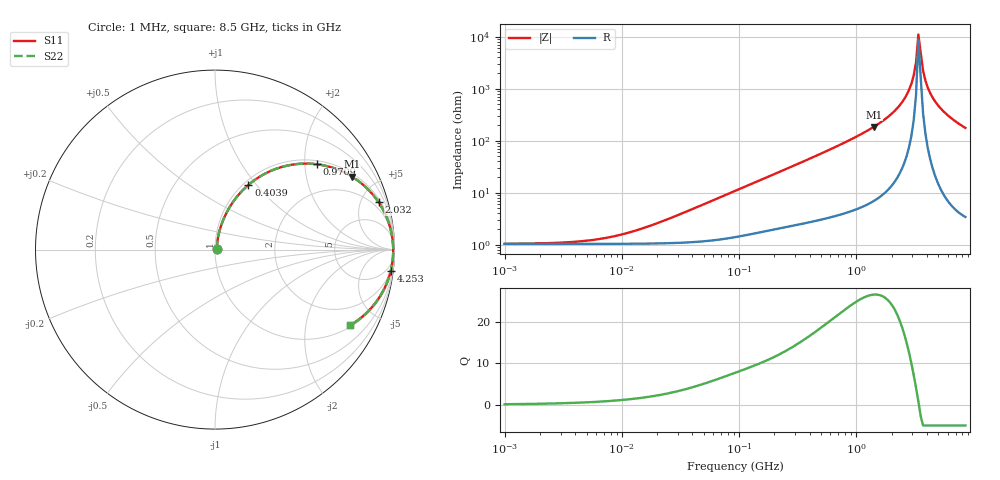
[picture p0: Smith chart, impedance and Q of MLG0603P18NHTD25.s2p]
! S-Parameter Data Generated by TDK Corporation
! Copyright(C) 2025 TDK Corporation.
! All Rights Reserved.
! TDK P/N: MLG0603P18NHTD25 (SMD / SMT Inductor (Coil))
! Property: L=18nH at 500MHz
! Size(LxWxT): 0.6x0.3x0.3mm
! Model Type: s2p (Touchstone File Format Version 1.0)
! Frequency: DC=Yes Start=1MHz Stop=8500MHz 198points Log-sweep
! Model Generated on Feb. 6, 2025
! Terms and conditions regarding TDK Simulation Models:
! 1)This simulation model is being provided solely for informational
!  purposes. Please refer to the specifications of the products in
!  terms of detailed characteristics of such products.
! 2)In no event shall TDK Corporation of any of its subsidiaries be
!  liable for any loss or damage arising, directly or indirectly,
!  from any information contained in this simulation model, including,
!  but not limited to loss or damages arising from any inaccuracies,
!  omissions or errors in connection with such information.
! 3)Any and all copyrights on this simulation model are owned by
!  TDK Corporation.  Duplication or redistribution of this simulation
!  model without prior written permission from TDK Corporation
!  is prohibited.
! 4)This simulation model is subject to any modification or change
!  without any prior notice.
! 5)Neither TDK Corporation nor any of its subsidiaries shall make any
!  warranty, express or implied, including but not limited to the
!  correctness, implied warranties of merchantability and fitness for
!  a particular purpose with respect to this simulation models.
! 6)The use of this simulation model shall be deemed to have consented
!  to the terms and conditions hereof.
! Port Assignments:
!  1 ---@@@--- 2
! Applicable Conditions:
!  Temperature = 25 degC
!  DC Bias Current = 0 A
!  Small Signal Operation
# Hz S MA R 50
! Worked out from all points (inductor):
!   197 points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, 1 MHz to 8.5 GHz, reference 50 ohm
!   read as one part in series: L = 18.8 nH near 27.76 MHz
!   highest Q = 26.5 at 1.405 GHz (marker M1), where L = 20.8 nH
!   self-resonance near 3.376 GHz
!   S11 on the Smith chart (normalised r, x): 1 MHz: 1.02, +0.00; 403.9 MHz: 1.05, +0.91; 970.9 MHz: 1.09, +2.31; 2.032 GHz: 1.29, +6.82; 4.253 GHz: 2, -17; 8.5 GHz: 1.07, -3.52
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1000000  0.01036 6.4  0.9897 -0.1  0.9897 -0.1  0.01036 6.4
4587603  0.01163 27.3  0.9897 -0.3  0.9897 -0.3  0.01163 27.3
9601846  0.01531 46.8  0.9896 -0.6  0.9896 -0.6  0.01531 46.8
2.10461e7  0.02685 65.5  0.9892 -1.4  0.9892 -1.4  0.02685 65.5
9.219544e7  0.1064 76.5  0.9807 -6.1  0.9807 -6.1  0.1064 76.5
2.216269e8  0.2404 71.4  0.9512 -13.9  0.9512 -13.9  0.2404 71.4
4.038753e8  0.4061 62.7  0.8898 -23.9  0.8898 -23.9  0.4061 62.7
4.229561e8  0.4218 61.7  0.8824 -24.9  0.8824 -24.9  0.4218 61.7
9.708683e8  0.7415 39.9  0.6415 -47.8  0.6415 -47.8  0.7415 39.9
1.404574e9  0.8652 28.0  0.47 -59.8  0.47 -59.8  0.8652 28.0
1.940355e9  0.9409 17.6  0.3025 -70.1  0.3025 -70.1  0.9409 17.6
2.032026e9  0.949 16.1  0.278 -71.5  0.278 -71.5  0.949 16.1
2.559585e9  0.9789 8.9  0.1546 -77.8  0.1546 -77.8  0.9789 8.9
2.939772e9  0.9888 4.6  0.08042 -79.7  0.08042 -79.7  0.9888 4.6
3.07866e9  0.9908 3.2  0.05574 -78.9  0.05574 -78.9  0.9908 3.2
3.224109e9  0.9922 1.7  0.03127 -74.6  0.03127 -74.6  0.9922 1.7
3.37643e9  0.9928 0.3  0.009041 -37.5  0.009041 -37.5  0.9928 0.3
3.703002e9  0.9923 -2.5  0.04475 78.8  0.04475 78.8  0.9923 -2.5
3.877948e9  0.991 -4.0  0.06947 80.6  0.06947 80.6  0.991 -4.0
4.253027e9  0.9864 -6.8  0.1193 80.1  0.1193 80.1  0.9864 -6.8
5.610304e9  0.9563 -15.6  0.2695 72.9  0.2695 72.9  0.9563 -15.6
8.5e9  0.862 -29.4  0.4904 59.5  0.4904 59.5  0.862 -29.4
